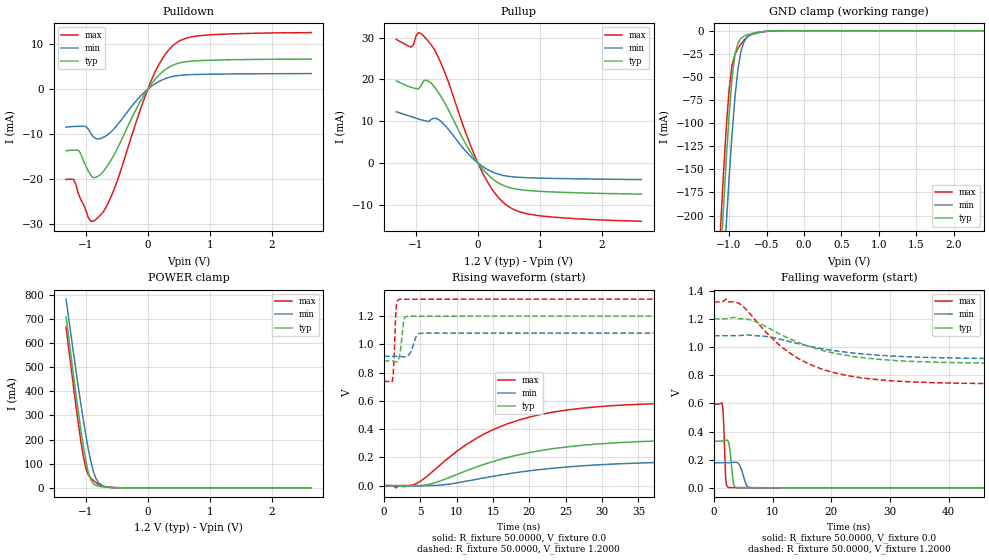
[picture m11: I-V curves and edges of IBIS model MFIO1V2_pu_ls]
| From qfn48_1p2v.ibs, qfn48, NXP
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[Model] MFIO1V2_pu_ls
|   Model MFIO1V2_pu_ls
| This model was characterised for following simulation conditions:
| External (pad) voltage:
|   - Typ: 1.2V,   - Min: 1.08V,   - Max: 1.32V
| Library cells for typ/min/max conditions are connected as defined below:
|  IO - External Pad
|  A - Core Input
|  EN - Output Buffer Enable
|  BOOST - vdde
|  EHS - gnd
|  ENZI - vdd
|  EPD - gnd
|  EPUN - gnd
|  ZI - NC
|  ZIF - NC
|  gnd - gnd
|  gnde - gnde
|  vdd - vdd
|  vdde - vdde
| All other pins connected to ground
Model_type I/O
Polarity   Non-Inverting
Enable   Active-Low
Vinl =   0.3600V
Vinh =   0.8400V
Vmeas =  0.6000V
Cref =   20.0000F
Rref =   1.0000M
Vref =   0.0V
C_comp   1.6368pF   1.5495pF   1.7160pF
|C_comp_pullup   0.8278pF   0.8638pF   0.7802pF
|C_comp_pulldown   0.5961pF   0.6350pF   0.5601pF
[Model Spec]
| variable   typ   min   max
Vinh   0.3600V   0.3240V   0.3960V
Vinl   0.8400V   0.7560V   0.9240V
Vmeas   0.6000V   0.5400V   0.6600V
[Temperature Range]   25.0000   0.1250k   -40.0000
[Voltage Range]   1.2000V   1.0800V   1.3200V
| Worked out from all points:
|   slope of the pulldown table from 0 to 0.18 V, typ, clamps not added: 58.2 ohm
|   slope of the pullup table from 0 to 0.18 V, typ, clamps not added: 59.4 ohm
|   GND clamp passes 1 mA (typ) near -0.56 V on its own axis
|   POWER clamp passes 1 mA (typ) near -0.54 V on its own axis
|   rising waveform, R_fixture 50.0000, V_fixture 0.0: 20-80 % time 14.4ns typ, 16.1ns min, 12.2ns max; typ from 0.001 V to 0.332 V
|   rising waveform, R_fixture 50.0000, V_fixture 1.2000: 20-80 % time 406ps typ, 667ps min, 259ps max; typ from 0.883 V to 1.2 V
|   falling waveform, R_fixture 50.0000, V_fixture 0.0: 20-80 % time 466ps typ, 793ps min, 299ps max; typ from 0.332 V to 0.001 V
|   falling waveform, R_fixture 50.0000, V_fixture 1.2000: 20-80 % time 12.6ns typ, 13.9ns min, 10.9ns max; typ from 1.2 V to 0.883 V
[Pulldown]
|Voltage   I(typ)   I(min)   I(max)
-1.32V    -13.65mA   -8.413mA   -20.02mA
-1.2V     -13.51mA   -8.286mA   -20.01mA
-1.12V    -13.55mA   -8.228mA   -23.23mA
-920mV    -19.16mA   -9.849mA   -29.29mA
-720mV    -18.27mA   -10.7mA    -27.21mA
-520mV    -13.92mA   -8.406mA   -21.33mA
-160mV    -3.727mA   -2.148mA   -6.154mA
80mV      1.535mA    840.4uA    2.681mA
280mV     4.299mA    2.312mA    7.674mA
480mV     5.684mA    2.989mA    10.42mA
960mV     6.383mA    3.3mA      11.99mA
2.64V     6.671mA    3.446mA    12.53mA
[Pullup]
|Voltage   I(typ)   I(min)   I(max)
-1.32V    19.64mA    12.26mA    29.6mA
-1.08V    18.12mA    11.13mA    27.73mA
-960mV    17.74mA    10.54mA    31.21mA
-840mV    19.83mA    10.07mA    29.84mA
-720mV    18.57mA    10.71mA    27.56mA
-520mV    13.94mA    8.794mA    21.09mA
-200mV    4.663mA    2.883mA    7.362mA
40mV      -771.3uA   -452.7uA   -1.28mA
240mV     -3.804mA   -2.171mA   -6.507mA
480mV     -5.732mA   -3.143mA   -10.26mA
1.04V     -6.794mA   -3.614mA   -12.68mA
2.64V     -7.439mA   -3.951mA   -13.93mA
[GND_clamp]
|Voltage   I(typ)   I(min)   I(max)
-1.32V    -596.2mA   -647.7mA   -564.2mA
-1.12V    -261.8mA   -329.6mA   -222.9mA
-1.08V    -200.1mA   -270.2mA   -162.2mA
-1.04V    -142.5mA   -213.4mA   -108mA
-1V       -91.69mA   -160.1mA   -64.43mA
-960mV    -51.28mA   -111.9mA   -37.39mA
-920mV    -25.2mA    -71.06mA   -25.22mA
-880mV    -12.91mA   -40.7mA    -18.88mA
-800mV    -5.723mA   -11.8mA    -10.08mA
-680mV    -2.609mA   -2.945mA   -3.568mA
-440mV    -184.2uA   -204.3uA   -227.8uA
2.64V     0A         0A         0A
[POWER_clamp]
|Voltage   I(typ)   I(min)   I(max)
-1.32V    708.1mA    782.2mA    666.5mA
-1.2V     465.4mA    558mA      418.6mA
-1.12V    311.6mA    414.7mA    262.8mA
-1.04V    171.5mA    279.6mA    128mA
-1V       111.6mA    216.9mA    80.27mA
-960mV    64.04mA    159.3mA    53.84mA
-920mV    33mA       108.8mA    40.21mA
-880mV    17.41mA    68.43mA    30.39mA
-840mV    10.75mA    40.17mA    22.03mA
-760mV    5.272mA    13.2mA     9.331mA
-440mV    212.2uA    284.9uA    247uA
2.64V     0A         0A         0A
[Ramp]
| variable   typ   min   max
dV/dt_r  0.1992/14.4262n   0.1068/16.1051n   0.3565/12.2258n
dV/dt_f  0.1901/12.5855n   98.6018m/13.9317n   0.3492/10.8859n
R_load = 50.0000
[Rising Waveform]
R_fixture= 50.0000
V_fixture= 0.0
V_fixture_min= 0.0
V_fixture_max= 0.0
|time   V(typ)   V(min)   V(max)
0s        575.5uV    578.6uV    543.8uV
1.683ns   664.8uV    652.9uV    -15.15mV
4.473ns   649.8uV    -3.694mV   15.46mV
6.773ns   17.28mV    1.315mV    104mV
11.21ns   103.6mV    30.81mV    287.3mV
16.88ns   198.1mV    82.76mV    435.9mV
21.68ns   249.8mV    115.5mV    505.3mV
27.07ns   284.9mV    140.2mV    547.5mV
45.07ns   325.2mV    171.6mV    588.9mV
100ns     332.5mV    178.5mV    594.8mV
[Rising Waveform]
R_fixture= 50.0000
V_fixture= 1.2000
V_fixture_min= 1.0800
V_fixture_max= 1.3200
|time   V(typ)   V(min)   V(max)
0s        883.2mV    915.7mV    738.1mV
1.166ns   881.8mV    915.9mV    744.4mV
1.362ns   879.8mV    916mV      866.5mV
1.679ns   876.6mV    915.3mV    1.263V
2.152ns   919.6mV    913.6mV    1.318V
2.75ns    1.171V     911.5mV    1.319V
3.316ns   1.199V     920mV      1.319V
4.556ns   1.199V     1.068V     1.319V
5.335ns   1.199V     1.079V     1.319V
100ns     1.2V       1.08V      1.32V
[Falling Waveform]
R_fixture= 50.0000
V_fixture= 0.0
V_fixture_min= 0.0
V_fixture_max= 0.0
|time   V(typ)   V(min)   V(max)
0s        332.5mV    178.5mV    594.8mV
1.413ns   332.8mV    178.5mV    588.5mV
1.613ns   334.5mV    178.5mV    478.3mV
2.005ns   339mV      178.4mV    53.58mV
2.548ns   309.5mV    179.3mV    2.904mV
3.302ns   30.31mV    182.3mV    2.199mV
4.03ns    2.21mV     178.2mV    2.279mV
5.549ns   1.723mV    17.33mV    1.812mV
6.564ns   1.628mV    1.877mV    1.499mV
100ns     575.5uV    578.7uV    543.8uV
[Falling Waveform]
R_fixture= 50.0000
V_fixture= 1.2000
V_fixture_min= 1.0800
V_fixture_max= 1.3200
|time   V(typ)   V(min)   V(max)
0s        1.2V       1.08V      1.32V
2.017ns   1.2V       1.08V      1.34V
4.477ns   1.2V       1.082V     1.304V
6.612ns   1.188V     1.081V     1.213V
10.48ns   1.108V     1.063V     1.038V
15.8ns    1.011V     1.01V      887.3mV
19.63ns   965.1mV    980mV      827.5mV
25.09ns   926mV      951.9mV    781.7mV
43.32ns   887.9mV    920.4mV    742.3mV
100ns     883.2mV    915.7mV    738.1mV
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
